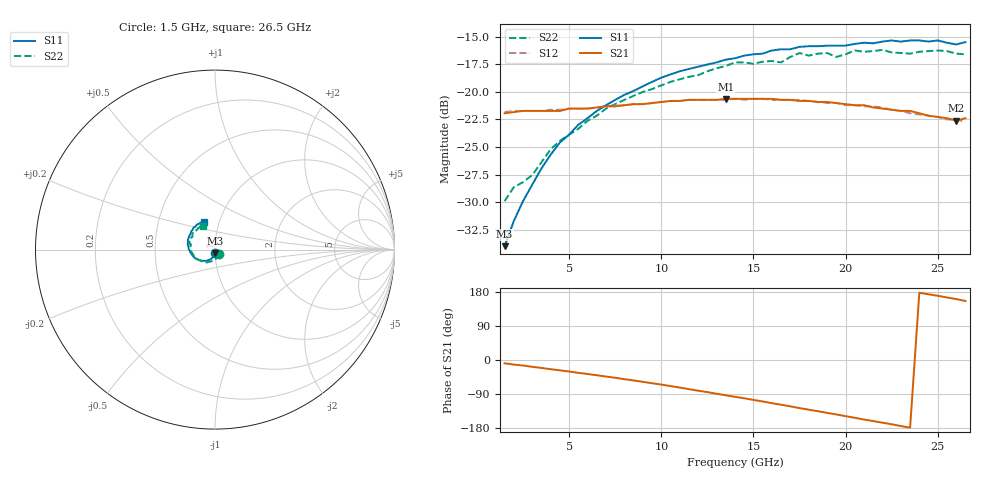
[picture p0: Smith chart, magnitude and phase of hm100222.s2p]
! HMMC-1002
! S-PARAMETERS at 22 dB attenuation setting. LAST UPDATED  07-06-99
# GHZ  S  MA  R  50
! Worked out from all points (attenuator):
!   51 points, 1.5 GHz to 26.5 GHz, reference 50 ohm
!   highest |S21| = -20.63 dB at 13.5 GHz (marker M1); lowest = -22.6 dB at 26 GHz (marker M2)
!   lowest |S11| = -34.0 dB at 1.5 GHz (marker M3), VSWR 1.04, Z = 49.9 - j2 ohm
!   |S11| at or under -10 dB: start of sweep to end of sweep
!   |S22| runs from -29.9 to -16.2 dB; largest |S21 - S12| = 0.0032
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1.5  0.02 -90.9  0.08 -8.6  0.081 -9.1  0.032 -45.2
2  0.026 -94.4  0.081 -12.1  0.082 -12.5  0.037 -55.3
2.5  0.032 -98.9  0.082 -14.6  0.082 -15.1  0.039 -66.5
3  0.038 -103.4  0.082 -18.0  0.082 -18.3  0.042 -77.1
3.5  0.045 -106.2  0.082 -21.0  0.082 -21.4  0.048 -81.9
4  0.052 -110.3  0.082 -24.2  0.083 -24.7  0.055 -88.0
4.5  0.059 -114.6  0.082 -27.3  0.083 -27.9  0.06 -94.6
6  0.076 -126.3  0.084 -36.9  0.084 -37.2  0.074 -113.4
7.5  0.092 -137.1  0.086 -46.8  0.087 -47.2  0.088 -126.3
10  0.116 -153.3  0.09 -64.9  0.09 -65.1  0.107 -147.1
13.5  0.14 -175.6  0.093 -93.0  0.092 -93.0  0.131 -173.7
14  0.142 -178.3  0.093 -97.2  0.093 -97.1  0.136 -175.9
16.5  0.156 166.3  0.092 -118.0  0.092 -117.9  0.136 168.3
17.5  0.16 161.5  0.091 -126.9  0.092 -126.6  0.15 162.3
18.5  0.161 155.8  0.09 -135.1  0.09 -135.2  0.149 159.1
19  0.162 152.9  0.09 -139.6  0.089 -139.4  0.15 154.4
19.5  0.162 149.4  0.089 -143.7  0.089 -143.7  0.144 150.8
20.5  0.165 144.7  0.087 -152.5  0.087 -152.2  0.154 143.8
22.5  0.171 133.5  0.083 -169.6  0.083 -169.4  0.151 136.6
25  0.171 118.6  0.077 169.5  0.077 169.5  0.154 119.6
26  0.164 114.6  0.074 160.8  0.075 162.0  0.149 117.3
26.5  0.168 111.9  0.076 155.7  0.073 156.6  0.148 116.1
